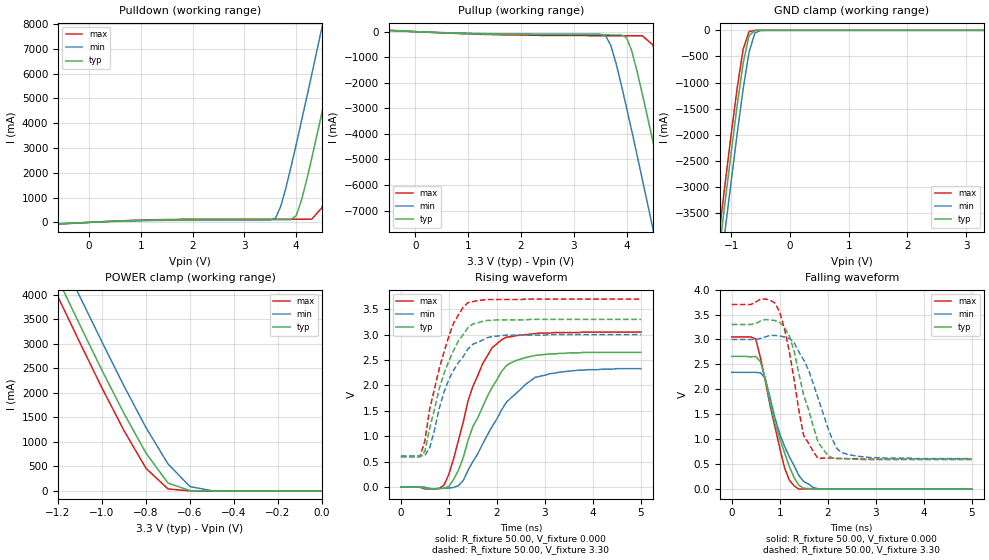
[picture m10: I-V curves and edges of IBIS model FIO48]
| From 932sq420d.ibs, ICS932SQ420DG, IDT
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|   Model FIO48
[Model]   FIO48
Model_type   I/O
Polarity   Non-Inverting
Enable   Active-High
Vinl =   0.80V
Vinh =   2.00V
Vmeas =   1.50V
C_comp   3.40pF   2.85pF   3.95pF
[Temperature Range]   27.00   70.00   0.000
[Voltage Range]   3.30V   3.00V   3.70V
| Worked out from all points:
|   slope of the pulldown table from 0 to 0.495 V, typ, clamps not added: 10.5 ohm
|   slope of the pullup table from 0 to 0.495 V, typ, clamps not added: 11.7 ohm
|   GND clamp passes 1 mA (typ) near -0.52 V on its own axis
|   POWER clamp passes 1 mA (typ) near -0.51 V on its own axis
|   rising waveform, R_fixture 50.00, V_fixture 0.000: 20-80 % time 726ps typ, 947ps min, 599ps max; typ from 0 V to 2.65 V
|   rising waveform, R_fixture 50.00, V_fixture 3.30: 20-80 % time 540ps typ, 569ps min, 492ps max; typ from 0.59 V to 3.3 V
|   falling waveform, R_fixture 50.00, V_fixture 0.000: 20-80 % time 454ps typ, 512ps min, 414ps max; typ from 2.66 V to 0 V
|   falling waveform, R_fixture 50.00, V_fixture 3.30: 20-80 % time 435ps typ, 525ps min, 341ps max; typ from 3.3 V to 0.59 V
[Pulldown]
| voltage   I(typ)   I(min)   I(max)
|  -3.30   0.000A   -0.29A   0.000A
|  -3.10   0.000A   0.000A   0.000A
|  -2.90   0.000A   0.000A   0.000A
|  -2.70   0.000A   0.000A   0.000A
|  -2.50   0.000A   0.000A   0.000A
|  -2.30   0.000A   0.000A   0.000A
|  -2.10   0.000A   0.000A   -10.00mA
|  -1.90   0.000A   0.000A   -10.00mA
|  -1.70   -3.00mA   -2.00mA   -2.00mA
|  -1.50   -3.00mA   -3.00mA   -3.00mA
|  -1.00   -8.00mA   -6.00mA   -9.00mA
|  -0.90   -12.00mA   -8.00mA   -15.00mA
|  -0.80   -21.50mA   -13.00mA   -33.00mA
|  -0.70   -49.90mA   -24.80mA   -68.49mA
-600mV    -59.67mA   -45.96mA   -65.12mA
3.6V      110mA      170mA      130mA
3.7V      110mA      640mA      130mA
3.8V      110mA      1.38A      130mA
4V        270mA      3.14A      130mA
4.1V      880mA      4.07A      130mA
4.3V      2.58A      5.96A      130mA
4.5V      4.45A      7.89A      600mA
4.7V      6.36A      9.83A      2.25A
4.9V      8.3A       11.78A     4.11A
5.3V      12.22A     15.71A     7.97A
6.6V      25.09A     28.59A     20.81A
[Pullup]
| voltage   I(typ)   I(min)   I(max)
|  -3.30   10.00mA   10.00mA   0.000A
|  -3.10   0.000A   10.00mA   0.000A
|  -2.90   0.000A   0.000A   0.000A
|  -2.70   10.00mA   0.000A   0.000A
|  -2.50   0.000A   0.000A   0.000A
|  -2.30   10.00mA   10.00mA   0.000A
|  -2.10   0.000A   10.00mA   0.000A
|  -1.90   0.000A   0.000A   0.000A
|  -1.70   3.00mA   3.00mA   2.00mA
|  -1.50   3.00mA   4.00mA   3.00mA
|  -1.00   7.00mA   6.00mA   10.00mA
|  -0.90   10.00mA   8.00mA   14.00mA
|  -0.80   18.40mA   12.00mA   28.20mA
|  -0.70   41.50mA   20.80mA   64.26mA
|  -0.60   56.82mA   40.37mA   63.47mA
-500mV    48.3mA     42.63mA    53.02mA
3.6V      -120mA     -150mA     -160mA
3.7V      -130mA     -520mA     -160mA
4V        -230mA     -2.97A     -160mA
4.1V      -760mA     -3.89A     -160mA
4.3V      -2.44A     -5.79A     -160mA
4.5V      -4.3A      -7.71A     -520mA
4.7V      -6.22A     -9.66A     -2.13A
4.9V      -8.16A     -11.62A    -3.99A
5.1V      -10.12A    -13.58A    -5.91A
5.3V      -12.08A    -15.56A    -7.85A
6.6V      -24.99A    -28.48A    -20.72A
[GND_clamp]
| voltage   I(typ)   I(min)   I(max)
-3.3V     -24.68A    -25.2A     -24.36A
-1.2V     -4.14A     -4.7A      -3.8A
-1.1V     -3.21A     -3.76A     -2.86A
-1V       -2.3A      -2.85A     -1.95A
-900mV    -1.42A     -1.96A     -1.09A
-800mV    -630mA     -1.12A     -360mA
-700mV    -100mA     -420mA     -22.65mA
-600mV    -3.69mA    -49.71mA   -740uA
-500mV    -170uA     -2.13mA    -87.52uA
3.3V      110pA      12.05uA    -12.59nA
[POWER_clamp]
| voltage   I(typ)   I(min)   I(max)
-3.3V     24.86A     25.41A     24.53A
-1.2V     4.32A      4.9A       3.96A
-1.1V     3.38A      3.96A      3.02A
-1V       2.46A      3.04A      2.1A
-900mV    1.58A      2.14A      1.23A
-800mV    770mA      1.29A      460mA
-700mV    160mA      550mA      40.14mA
-600mV    6.42mA     88.58mA    710uA
-500mV    150uA      4.03mA     28.41uA
0V        110pA      1.99nA     120pA
[Ramp]
| variable   typ   min   max
dV/dt_r   1.59/0.73n   1.40/0.92n   1.83/0.60n
dV/dt_f   1.63/0.43n   1.43/0.51n   1.86/0.36n
R_load = 50.00
[Rising Waveform]
R_fixture = 50.00
V_fixture = 0.000
V_fixture_min = 0.000
V_fixture_max = 0.000
| time   V(typ)   V(min)   V(max)
0s        240uV      190uV      310uV
900ps     -23.2mV    -25.24mV   38.3mV
1ns       9.92mV     -21.34mV   250mV
1.2ns     330mV      26.23mV    920mV
1.5ns     1.19V      500mV      1.98V
1.9ns     1.96V      1.19V      2.74V
2.1ns     2.28V      1.52V      2.9V
2.3ns     2.45V      1.76V      2.96V
2.8ns     2.59V      2.16V      3.02V
5ns       2.65V      2.33V      3.05V
[Rising Waveform]
R_fixture = 50.00
V_fixture = 3.30
V_fixture_min = 3.00
V_fixture_max = 3.70
| time   V(typ)   V(min)   V(max)
0s        590mV      610mV      600mV
400ps     590mV      610mV      600mV
500ps     700mV      620mV      910mV
600ps     1.15V      770mV      1.53V
800ps     1.94V      1.55V      2.33V
1ns       2.48V      2.12V      2.97V
1.1ns     2.69V      2.3V       3.23V
1.4ns     3.14V      2.72V      3.63V
2.2ns     3.29V      2.99V      3.69V
5ns       3.3V       3V         3.7V
[Falling Waveform]
R_fixture = 50.00
V_fixture = 0.000
V_fixture_min = 0.000
V_fixture_max = 0.000
| time   V(typ)   V(min)   V(max)
0s        2.66V      2.34V      3.05V
500ps     2.66V      2.34V      3.01V
600ps     2.55V      2.33V      2.63V
700ps     2.21V      2.22V      2.17V
900ps     1.32V      1.43V      1.25V
1.1ns     730mV      860mV      430mV
1.2ns     450mV      650mV      180mV
1.4ns     74.91mV    270mV      -2.6mV
1.8ns     3.48mV     7.51mV     3.51mV
5ns       240uV      210uV      320uV
[Falling Waveform]
R_fixture = 50.00
V_fixture = 3.30
V_fixture_min = 3.00
V_fixture_max = 3.70
| time   V(typ)   V(min)   V(max)
0s        3.3V       3V         3.7V
900ps     3.38V      3.08V      3.73V
1ns       3.34V      3.07V      3.55V
1.2ns     3.07V      3.02V      2.76V
1.3ns     2.77V      2.94V      2.2V
1.5ns     1.88V      2.59V      1.07V
1.8ns     940mV      1.82V      610mV
2.1ns     620mV      990mV      620mV
2.3ns     610mV      730mV      610mV
5ns       590mV      610mV      600mV
